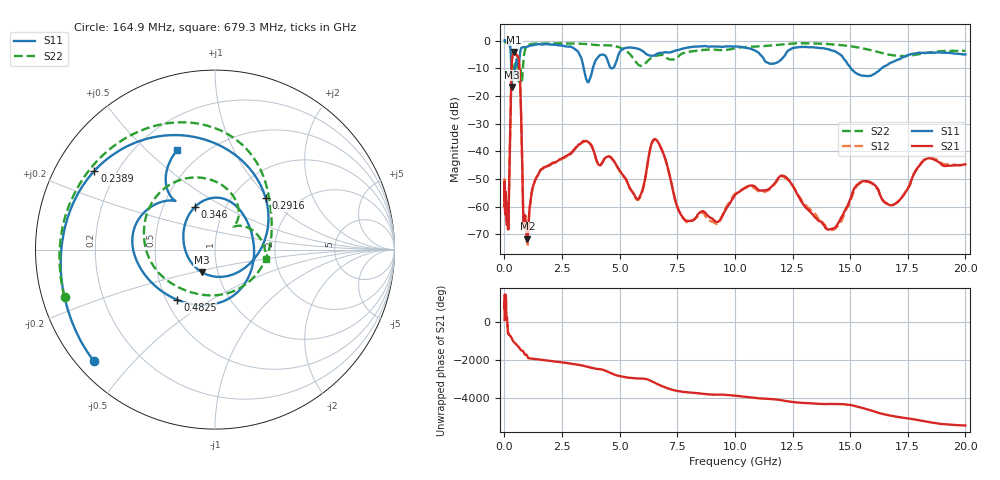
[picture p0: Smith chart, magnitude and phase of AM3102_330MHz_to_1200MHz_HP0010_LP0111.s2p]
! Date/Time: Tue, Sep 11, 2018 5:10 PM
! Network Analyzer: Agilent Technologies E8362B Rev: A.07.50.63
! Sweep from 0.010 to 20.000 GHz, 1601 Points, Sweep Type: LOG
! Power Supply: 4.949 V, 0.001 A
# Hz S DB R 50
!freq MagS11 AngS11 MagS21 AngS21 MagS12 AngS12 MagS22 AngS22
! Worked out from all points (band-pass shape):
!   1601 points, 10 MHz to 20 GHz, reference 50 ohm
!   highest |S21| = -4.12 dB at 422.4 MHz (marker M1); lowest = -71.5 dB at 998.1 MHz (marker M2)
!   |S21| within 3 dB of the highest: 328 MHz to 626.4 MHz (298.4 MHz wide, 62.5 % of centre)
!   lowest |S11| = -16.7 dB at 319.2 MHz (marker M3), VSWR 1.34, Z = 41.9 - j10.8 ohm
!   |S11| at or under -10 dB: 297.6 MHz to 467.2 MHz (169.6 MHz wide, 44.3 % of centre); 3.439 GHz to 3.836 GHz (397 MHz wide, 10.9 % of centre); 15.03 GHz to 16.37 GHz (1.345 GHz wide, 8.57 % of centre)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
!   |S22| runs from -15.7 to -0.2 dB; largest |S21 - S12| = 0.011
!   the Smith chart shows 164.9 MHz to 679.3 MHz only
!   S11 on the Smith chart (normalised r, x): 164.9 MHz: 0.05, -0.39; 238.9 MHz: 0.12, +0.29; 291.6 MHz: 1.40, +0.96; 346 MHz: 0.72, +0.37; 482.5 MHz: 0.57, -0.36; 679.3 MHz: 0.37, +0.63
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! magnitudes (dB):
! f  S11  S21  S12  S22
! 10 MHz  0.0  -51.5  -51.6  -0.2
! 35.55 MHz  0.0  -61.0  -60.7  -0.4
! 126.4 MHz  -0.4  -64.8  -65.0  -0.9
! 164.9 MHz  -0.7  -66.2  -63.4  -1.1
! 238.9 MHz  -1.9  -38.5  -38.6  -1.7
! 291.6 MHz  -7.9  -15.5  -15.6  -3.8
! 319.2 MHz  -16.7  -8.3  -8.3  -7.2
! 346 MHz  -11.6  -5.8  -5.9  -10.1
! 422.4 MHz  -12.9  -4.1  -4.2  -10.4
! 447.2 MHz  -11.2  -4.2  -4.3  -9.0
! 482.5 MHz  -9.1  -4.5  -4.6  -7.8
! 679.3 MHz  -4.5  -14.3  -14.4  -10.8
! 833.3 MHz  -2.4  -66.3  -66.3  -6.6
! 998.1 MHz  -2.2  -71.5  -74.3  -1.9
! 1.59 GHz  -1.4  -46.6  -46.6  -1.0
! 3.582 GHz  -14.5  -36.3  -36.3  -1.3
! 5.652 GHz  -2.7  -55.9  -56.0  -7.1
! 6.58 GHz  -5.0  -35.8  -35.9  -5.5
! 7.882 GHz  -2.7  -65.1  -65.5  -4.3
! 12.03 GHz  -6.6  -48.8  -49.2  -1.4
! 14.14 GHz  -3.4  -68.1  -68.5  -1.3
! 20 GHz  -5.0  -44.7  -45.1  -3.7
